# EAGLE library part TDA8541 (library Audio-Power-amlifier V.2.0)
The TDA8541(T) is a one channel audio power amplifier for an output power of 1 W with an 8 Ω load at a 5 V supply. The circuit contains a BTL amplifier with a complementary PNP-NPN output stage and standby/mute logic. The TDA8541T comes in an 8 pin SO package and the TDA8541 in an 8 pin DIP package.
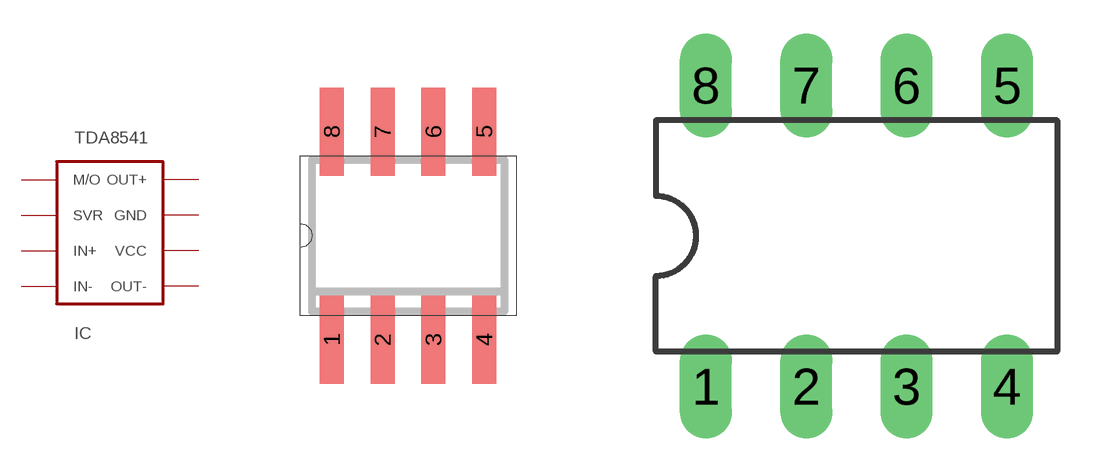
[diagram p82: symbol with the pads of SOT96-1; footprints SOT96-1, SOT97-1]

Designator prefix IC

## TDA8541SO8  [SOT96-1]
1  M/O  in
2  SVR  in
3  IN+  in
4  IN-  in
5  OUT-  out
6  VCC  pwr
7  GND  pwr
8  OUT+  out

## TDA8541DIL8  [SOT97-1]
Pads as for SOT96-1

## Footprint SOT96-1 (pad centres in mm)
Small Outline Narrow Plastic Gull Wing 150-mil body, package type SN
smd 0.6 x 2.2: 1 -1.905,-2.6; 2 -0.635,-2.6; 3 0.635,-2.6; 4 1.905,-2.6; 5 1.905,2.6; 6 0.635,2.6; 7 -0.635,2.6; 8 -1.905,2.6

## Footprint SOT97-1 (pad centres in mm)
Dual In Line Package
drill 0.813 long: 1 -3.81,-3.81; 2 -1.27,-3.81; 3 1.27,-3.81; 4 3.81,-3.81; 5 3.81,3.81; 6 1.27,3.81; 7 -1.27,3.81; 8 -3.81,3.81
